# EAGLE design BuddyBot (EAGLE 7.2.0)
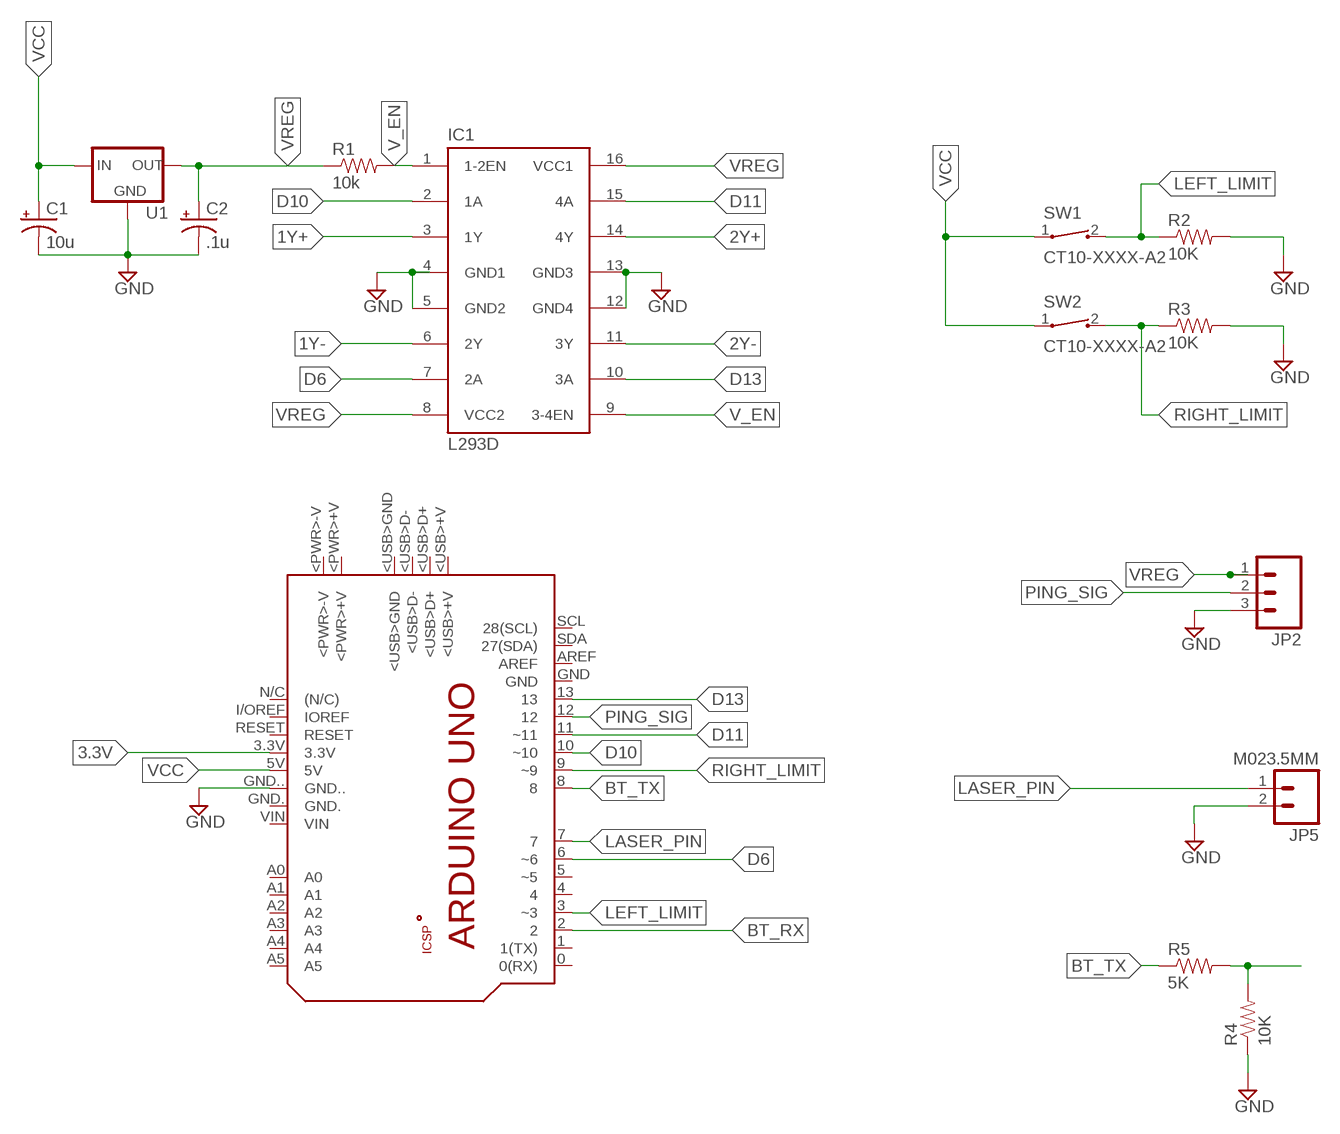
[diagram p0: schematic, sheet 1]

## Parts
C1  10u  CPOL-USE3.5-8  [E3,5-8]
C2  .1u  CPOL-USE3.5-8  [E3,5-8]
IC1  L293D  [DIL16]
JP2  M03-SCREW-5MM  [SCREWTERMINAL-5MM-3]
JP5  M023.5MM  [SCREWTERMINAL-3.5MM-2]
PCB1  ARDUINO_UNO  [ARDUINO_UNO]
R1  10k  RESISTORAXIAL-0.3  [AXIAL-0.3]
R2  10K  RESISTORAXIAL-0.3  [AXIAL-0.3]
R3  10K  RESISTORAXIAL-0.3  [AXIAL-0.3]
R4  10K  RESISTORAXIAL-0.3  [AXIAL-0.3]
R5  5K  RESISTORAXIAL-0.3  [AXIAL-0.3]
SW1  CT10-XXXX-A2  [CT10-XXXX-A2]
SW2  CT10-XXXX-A2  [CT10-XXXX-A2]
U1  V_REG_78XX-TO-220  [TO-220-ALT]

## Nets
1Y+: IC1.3(1Y)
1Y-: IC1.6(2Y)
2Y+: IC1.14(4Y)
2Y-: IC1.11(3Y)
3.3V: PCB1.3.3V
BT_RX: PCB1.2
BT_TX: PCB1.8 R5.P$1
D6: IC1.7(2A) PCB1.6(~6)
D10: IC1.2(1A) PCB1.10(~10)
D11: IC1.15(4A) PCB1.11(~11)
D13: IC1.10(3A) PCB1.13
GND: C1.- C2.- IC1.4(GND1) IC1.5(GND2) IC1.12(GND4) IC1.13(GND3) JP2.3 JP5.2 PCB1.GND.. R2.P$2 R3.P$2 R4.P$1 U1.GND
LASER_PIN: JP5.1 PCB1.7
LEFT_LIMIT: PCB1.3(~3) R2.P$1 SW1.2
N$5: R4.P$2 R5.P$2
PING_SIG: JP2.2 PCB1.12
RIGHT_LIMIT: PCB1.9(~9) R3.P$1 SW2.2
V_EN: IC1.1(1-2EN) IC1.9(3-4EN) R1.P$2
VCC: C1.+ PCB1.5V SW1.1 SW2.1 U1.IN
VREG: C2.+ IC1.8(VCC2) IC1.16(VCC1) JP2.1 R1.P$1 U1.OUT
Unconnected: PCB1.0(0(RX)) PCB1.1(1(TX)) PCB1.4 PCB1.5(~5) PCB1.+5V PCB1.<PWR>+V PCB1.<PWR>-V PCB1.<USB>+V PCB1.<USB>D+ PCB1.<USB>D- PCB1.<USB>GND PCB1.A0 PCB1.A1 PCB1.A2 PCB1.A3 PCB1.A4 PCB1.A5 PCB1.AREF PCB1.GND PCB1.GND. PCB1.GND_ PCB1.I/OREF(IOREF) PCB1.MISO PCB1.MOSI PCB1.N/C((N/C)) PCB1.RESET PCB1.RESET. PCB1.SCK PCB1.SCL(28(SCL)) PCB1.SDA(27(SDA)) PCB1.VIN

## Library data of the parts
C1 C2 = adafruit:CPOL-US: POLARIZED CAPACITOR, American symbol
IC1 = st-microelectronics:L293D: PUSH-PULL 4 CHANNEL DRIVER; MPN: L293D; OC_FARNELL: 9589619; OC_NEWARK: 56P8249
JP2 = SparkFun-Connectors:M03: Header 3 Standard 3-pin 0.1" header. Use with straight break away headers (SKU : PRT-00116), right angle break away headers (PRT-00553), swiss pins (PRT-00743), machine pins (PRT-00117), and female headers (PRT-00115). Molex polarized connector foot print use with SKU : PRT-08232 with associated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; STOREFRONT_ID: PRT-08433
JP5 = SparkFun-Connectors:M02: Standard 2-pin 0.1" header. Use with; PROD_ID: CONN-08399
PCB1 = E14_Arduino_revB:ARDUINO_UNO: Device for representing an Arduino Uno board with a footprint in an EAGLE design. Created by Dave Young for Element14. More EAGLE documentation at: http://www.element14.com/community/community/knode/cadsoft_eagle
R1-R5 = SparkFun-Resistors:RESISTOR: Resistor
SW1 SW2 = switch-coto:CT10-XXXX-: CT10 Series Molded Switch
U1 = SparkFun-PowerIC:V_REG_78XX: Voltage Regulator Standard 78xx regulator. IGO (Input Ground Output). Spark Fun Electronics SKU : COM-00107; PROD_ID: VREG-08450; SF_ID: COM-00107

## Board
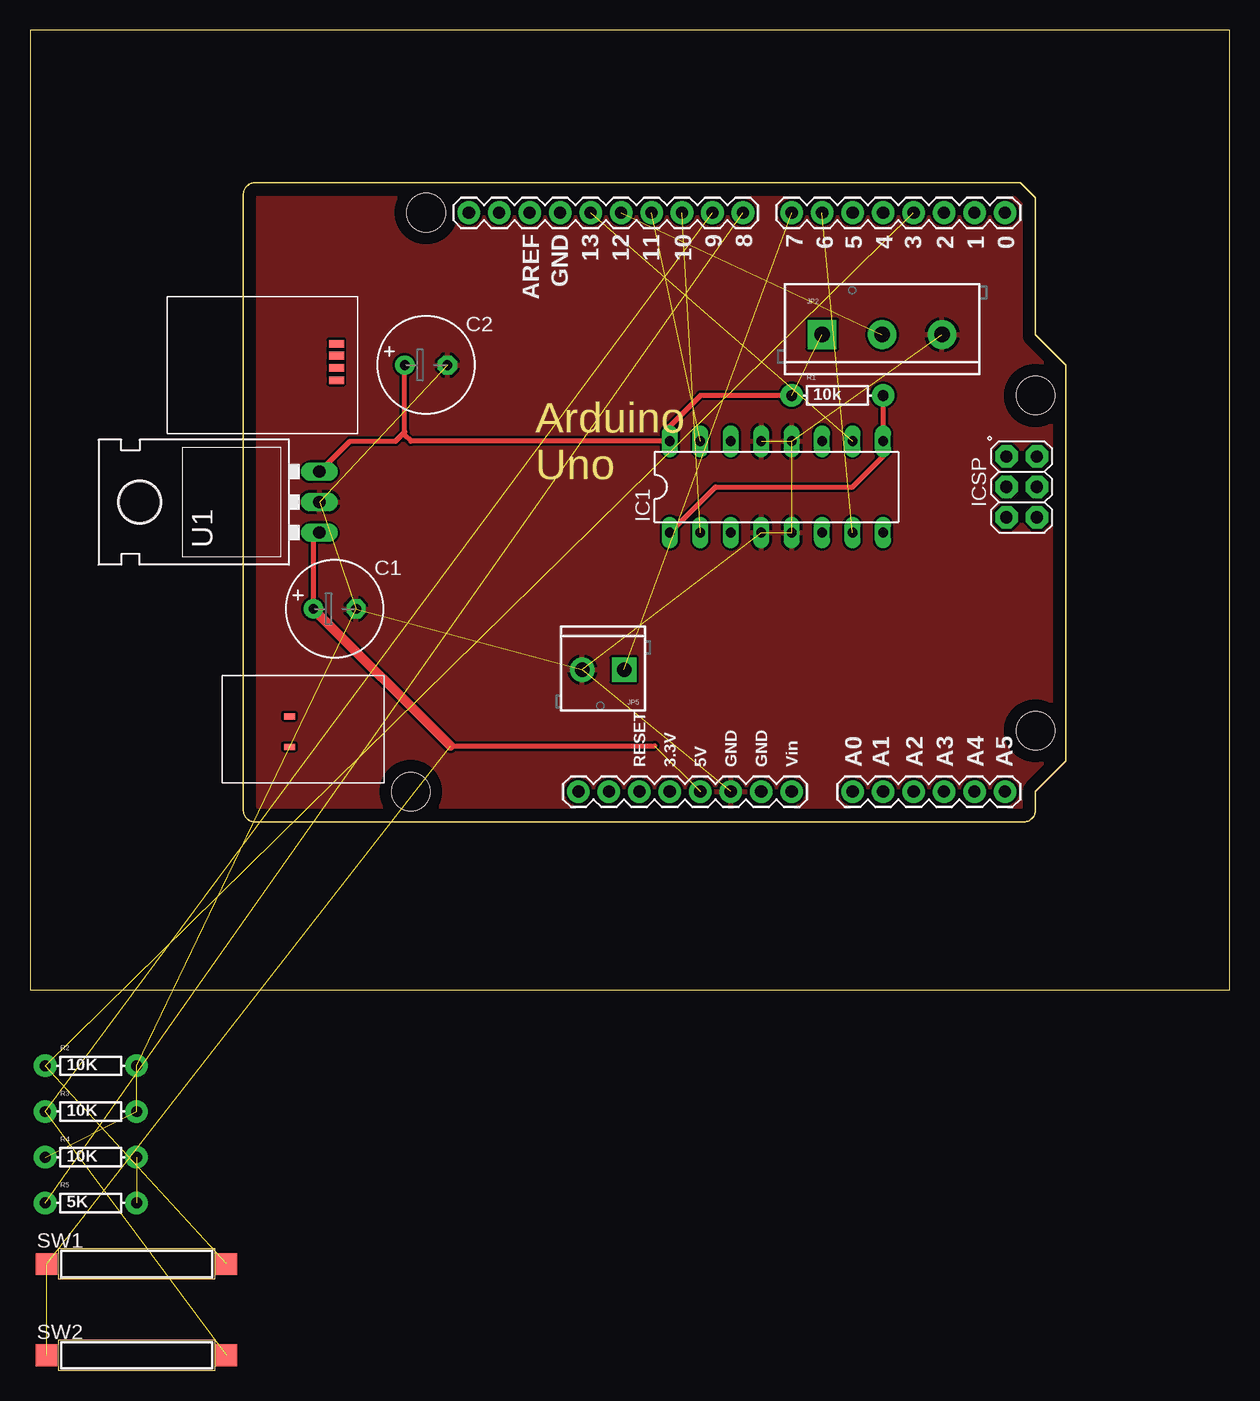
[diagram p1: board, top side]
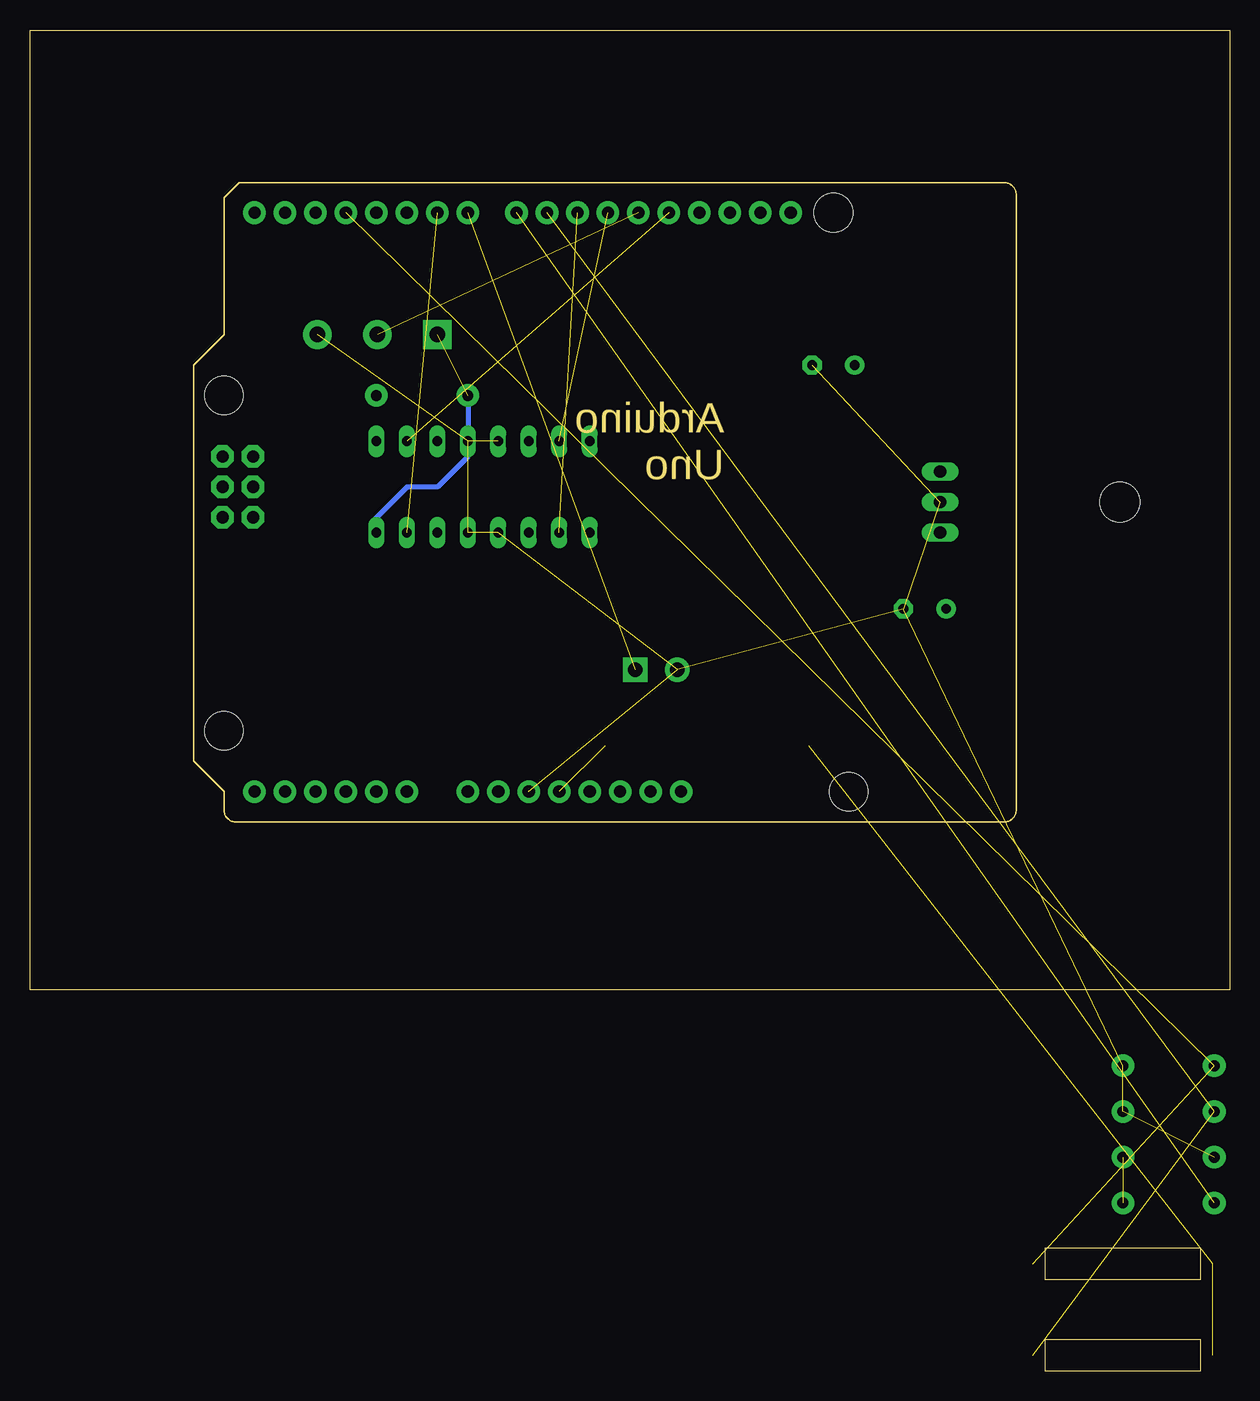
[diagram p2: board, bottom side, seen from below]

Size 100 x 111.78 mm. Coordinates in mm from the lower left corner, seen from the top.
Outline: 0,31.78 100,31.78 100,111.78 0,111.78 0,31.78
Copper layers (1*16): Top 0.035mm / dielectric 1.5mm / Bottom 0.035mm
Design rules "default": minimum track width 10mil, minimum drill 24mil, track to track 8mil, track to pad 8mil, pad to pad 8mil, via to via 8mil, smd to smd 8mil, copper to edge 40mil, drill to drill 8mil, minimum pad ring 10mil, minimum via ring 8mil, stop-mask expansion 4mil, vias tented up to drill 0mil, thermal gap 10mil

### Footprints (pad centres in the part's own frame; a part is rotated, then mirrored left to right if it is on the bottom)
E3,5-8 = drill 0.813 pad 1.6: + -1.778,0 | drill 0.813 pad 1.6 octagon: - 1.778,0
DIL16 = drill 0.813 long: 1 -8.89,-3.81; 2 -6.35,-3.81; 3 -3.81,-3.81; 4 -1.27,-3.81; 5 1.27,-3.81; 6 3.81,-3.81; 7 6.35,-3.81; 8 8.89,-3.81; 9 8.89,3.81; 10 6.35,3.81; 11 3.81,3.81; 12 1.27,3.81; 13 -1.27,3.81; 14 -3.81,3.81; 15 -6.35,3.81; 16 -8.89,3.81
SCREWTERMINAL-5MM-3 = drill 1.3 pad 2.413 square: 1 0,0 | drill 1.3 pad 2.413: 2 5,0; 3 10,0
SCREWTERMINAL-3.5MM-2 = drill 1.2 pad 2.032 square: 1 0,0 | drill 1.2 pad 2.032: 2 3.5,0
ARDUINO_UNO = drill 1.016 pad 1.88: 0 63.5,50.8; 1 60.96,50.8; 2 58.42,50.8; 3 55.88,50.8; 3.3V 35.56,2.54; 4 53.34,50.8; 5 50.8,50.8; 5V 38.1,2.54; 6 48.26,50.8; 7 45.72,50.8; 8 41.656,50.8; 9 39.116,50.8; 10 36.576,50.8; 11 34.036,50.8; 12 31.496,50.8; 13 28.956,50.8; A0 50.8,2.54; A1 53.34,2.54; A2 55.88,2.54; A3 58.42,2.54; A4 60.96,2.54; A5 63.5,2.54; AREF 23.876,50.8; GND 26.416,50.8; GND. 43.18,2.54; GND.. 40.64,2.54; I/OREF 30.48,2.54; N/C 27.94,2.54; RESET 33.02,2.54; SCL 18.796,50.8; SDA 21.336,50.8; VIN 45.72,2.54 | drill 1.016 pad 1.88 octagon: +5V 66.167,30.48; GND_ 66.167,25.4; MISO 63.627,30.48; MOSI 66.167,27.94; RESET. 63.627,25.4; SCK 63.627,27.94 | smd 1.016 x 0.508: <PWR>+V 3.861,8.814; <PWR>-V 3.861,6.274 | smd 1.27 x 0.635: <USB>+V 7.772,39.878; <USB>D+ 7.772,38.887; <USB>D- 7.772,37.871; <USB>GND 7.772,36.83 | hole 3.2: 66.04,7.62; 66.04,35.56; 15.24,50.8; 13.97,2.54
AXIAL-0.3 = drill 0.9 pad 1.88: P$1 -3.81,0; P$2 3.81,0
CT10-XXXX-A2 = smd 1.8 x 1.8: 1 -7.5,0; 2 7.5,0
TO-220-ALT = drill 1.016 long: GND 0,-3.81; IN -2.54,-3.81; OUT 2.54,-3.81 | hole 3.302: 0,11.176

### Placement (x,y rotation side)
C1  25.4,63.53 0 top
C2  33.02,83.85 0 top
IC1  62.23,73.69 0 top
JP2  66.04,86.39 0 top
JP5  49.53,58.45 180 top
PCB1  17.78,45.75 0 top
R1  67.31,81.31 0 top
R2  5.08,25.43 0 top
R3  5.08,21.62 0 top
R4  5.08,17.81 0 top
R5  5.08,14 0 top
SW1  8.89,8.92 0 top
SW2  8.89,1.3 0 top
U1  20.32,72.42 90 top

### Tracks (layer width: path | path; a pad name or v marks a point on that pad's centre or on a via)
BT_TX  (1 unrouted)
D6  (1 unrouted)
D10  (1 unrouted)
D11  (1 unrouted)
D13  (1 unrouted)
GND  (12 unrouted)
  pour Top: 16.51,100.36 16.51,44.48 87.63,44.48 87.63,100.36
LASER_PIN  (1 unrouted)
LEFT_LIMIT  (2 unrouted)
N$5  (1 unrouted)
PING_SIG  (1 unrouted)
RIGHT_LIMIT  (2 unrouted)
V_EN
  Top 0.406: IC1.1 57.15,73.69 68.58,73.69 71.12,76.23 IC1.9 R1.P$2
VCC  (3 unrouted)
  Top 0.406: 35.05,52.1 52.07,52.1 | U1.IN 23.62,69.37 C1.+
  Top 0.813: C1.+ 35.05,52.1
VREG  (1 unrouted)
  Top 0.406: U1.OUT 26.67,77.5 30.48,77.5 31.24,78.26 | 31.24,78.26 C2.+ | R1.P$1 55.88,81.31 53.34,78.77 IC1.16 31.75,77.5 31.24,78.01 31.24,78.26
  Bottom 0.406: R1.P$1 63.5,76.23 66.04,73.69 68.58,73.69 71.12,71.15 IC1.8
